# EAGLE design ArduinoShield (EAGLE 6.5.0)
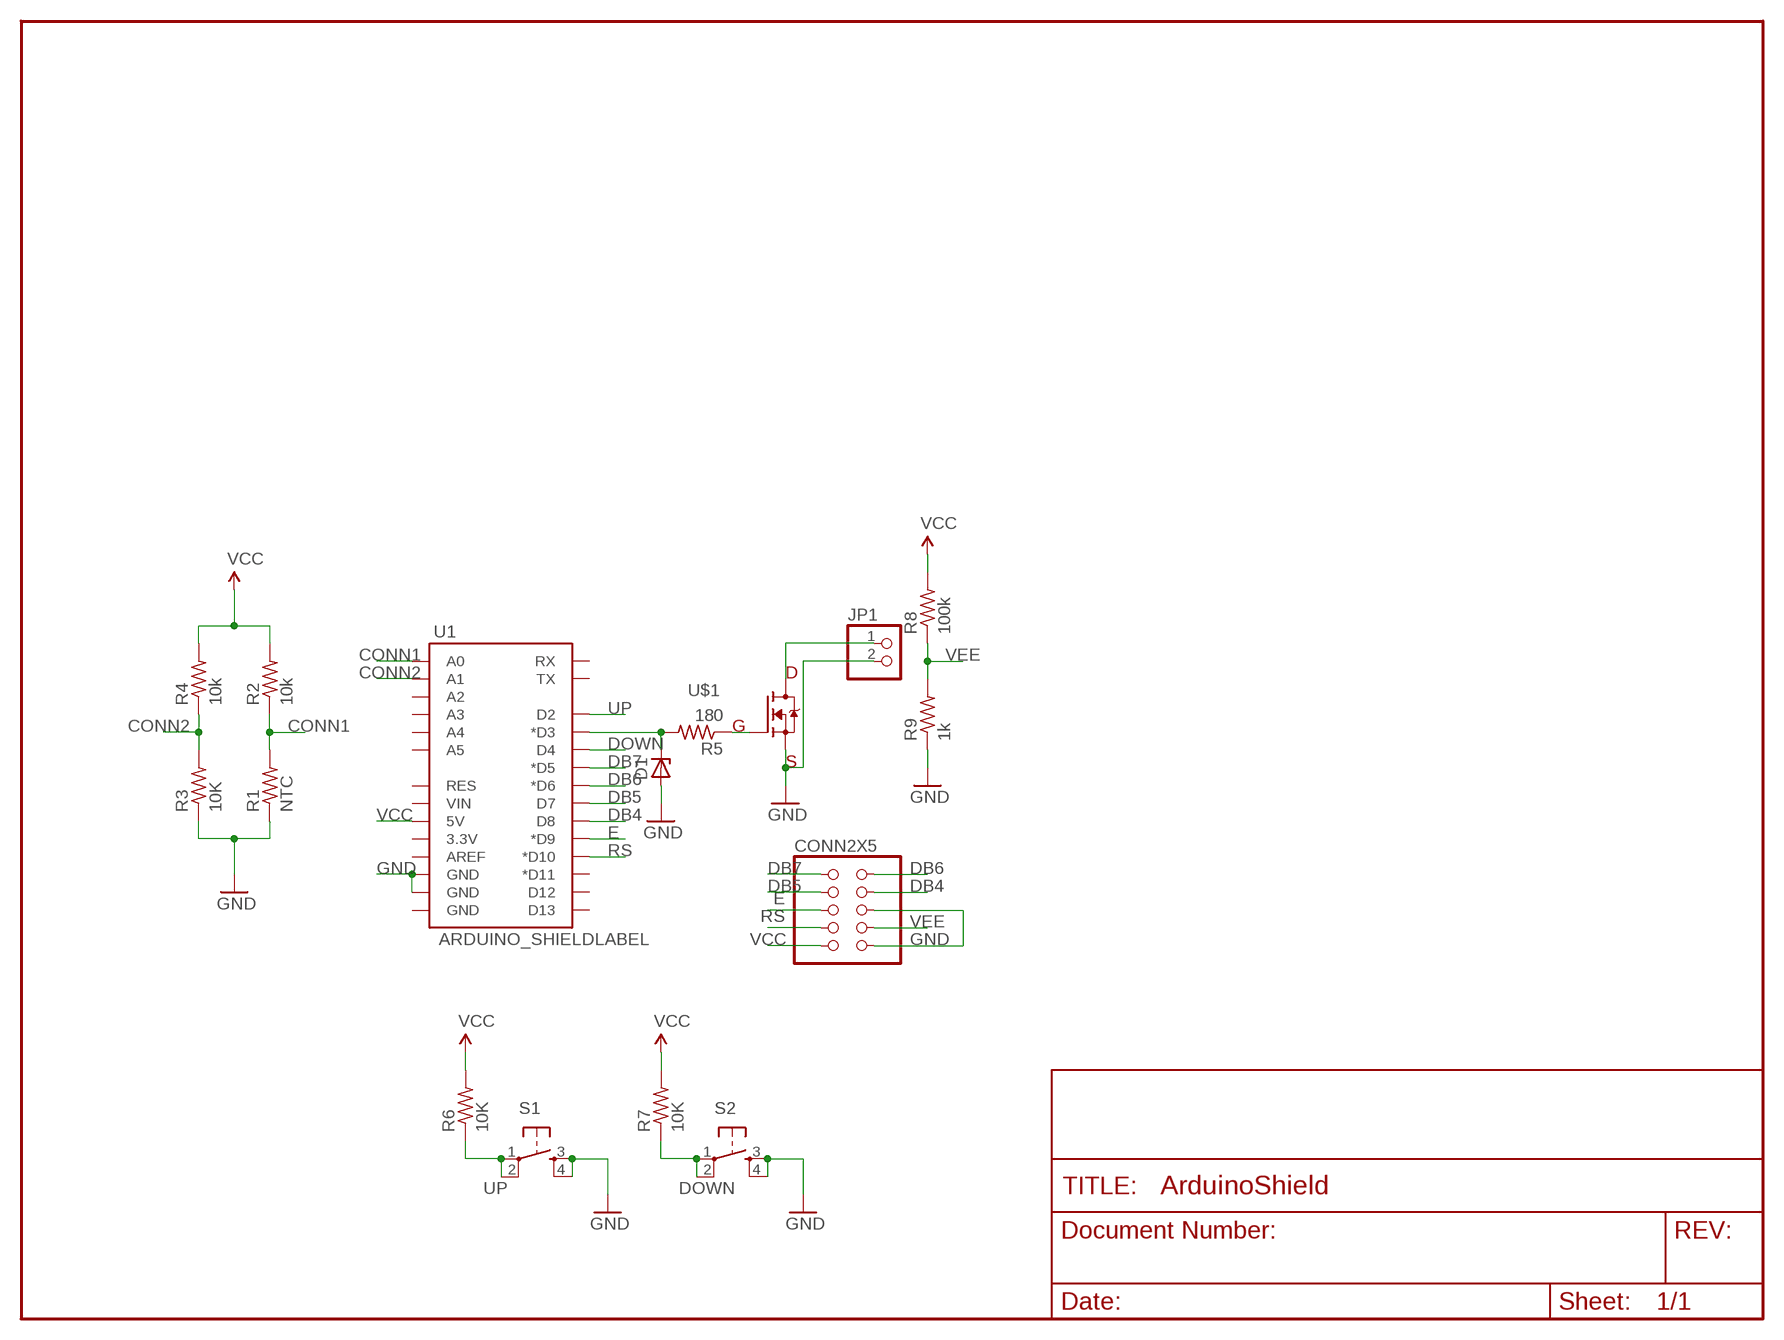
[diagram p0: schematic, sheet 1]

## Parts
CONN2X5  CONN2X05  [2X05SMD]
D1  ZENER_DIODESOD123  [SOD123]
JP1  PINHD-1X2  [1X02]
R1  NTC  RESISTOR1206  [1206]
R2  10k  RESISTOR1206  [1206]
R3  10K  RESISTOR1206  [1206]
R4  10k  RESISTOR1206  [1206]
R5  180  RESISTOR1206  [1206]
R6  10K  RESISTOR1206  [1206]
R7  10K  RESISTOR1206  [1206]
R8  100k  RESISTOR1206  [1206]
R9  1k  RESISTOR1206  [1206]
S1  6MM_SWITCH6MM_SWITCH  [6MM_SWITCH]
S2  6MM_SWITCH6MM_SWITCH  [6MM_SWITCH]
U1  ARDUINO_SHIELDLABEL  [DUEMILANOVE_SHIELD]
U$1  N-MOSFETTO-252  [N-MOSFET]

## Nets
CONN1: R1.2 R2.1 U1.A0
CONN2: R3.2 R4.1 U1.A1
DB4: CONN2X5.7(DB4) U1.D8
DB5: CONN2X5.8(DB5) U1.D7
DB6: CONN2X5.9(DB6) U1.D6(*D6)
DB7: CONN2X5.10(DB7) U1.D5(*D5)
DOWN: R7.1 S2.1(P) S2.2(P1) U1.D4
E: CONN2X5.6(E) U1.D9(*D9)
GND: CONN2X5.1(GND) CONN2X5.5(R/W) D1.ANODE JP1.2 R1.1 R3.1 R9.1 S1.3(S) S1.4(S1) S2.3(S) S2.4(S1) U1.GND@1(GND) U1.GND@2(GND) U$1.2(S)
N$1: D1.CATHODE R5.2 U1.D3(*D3)
N$2: R5.1 U$1.1(G)
N$3: JP1.1 U$1.3(D)
RS: CONN2X5.4(RS) U1.D10(*D10)
UP: R6.1 S1.1(P) S1.2(P1) U1.D2
VCC: CONN2X5.2(VCC) R2.2 R4.2 R6.2 R7.2 R8.2 U1.5V
VEE: CONN2X5.3(VEE) R8.1 R9.2
Unconnected: U1.3.3V U1.A2 U1.A3 U1.A4 U1.A5 U1.AREF U1.D11(*D11) U1.D12 U1.D13 U1.GND@0(GND) U1.RES U1.RX U1.TX U1.VIN

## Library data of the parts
CONN2X5 = 01_ng:CONN2X05
D1 = 01_ng:ZENER_DIODE: zener diode
JP1 = pinhead:PINHD-1X2: PIN HEADER
R1-R9 = 01_ng:RESISTOR
S1 S2 = 01_ng:6MM_SWITCH: OMRON SWITCH
U1 = 01_SparkFun:ARDUINO_SHIELD
U$1 = 01_Ali:N-MOSFET

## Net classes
0 default: clearance 0.205 mm

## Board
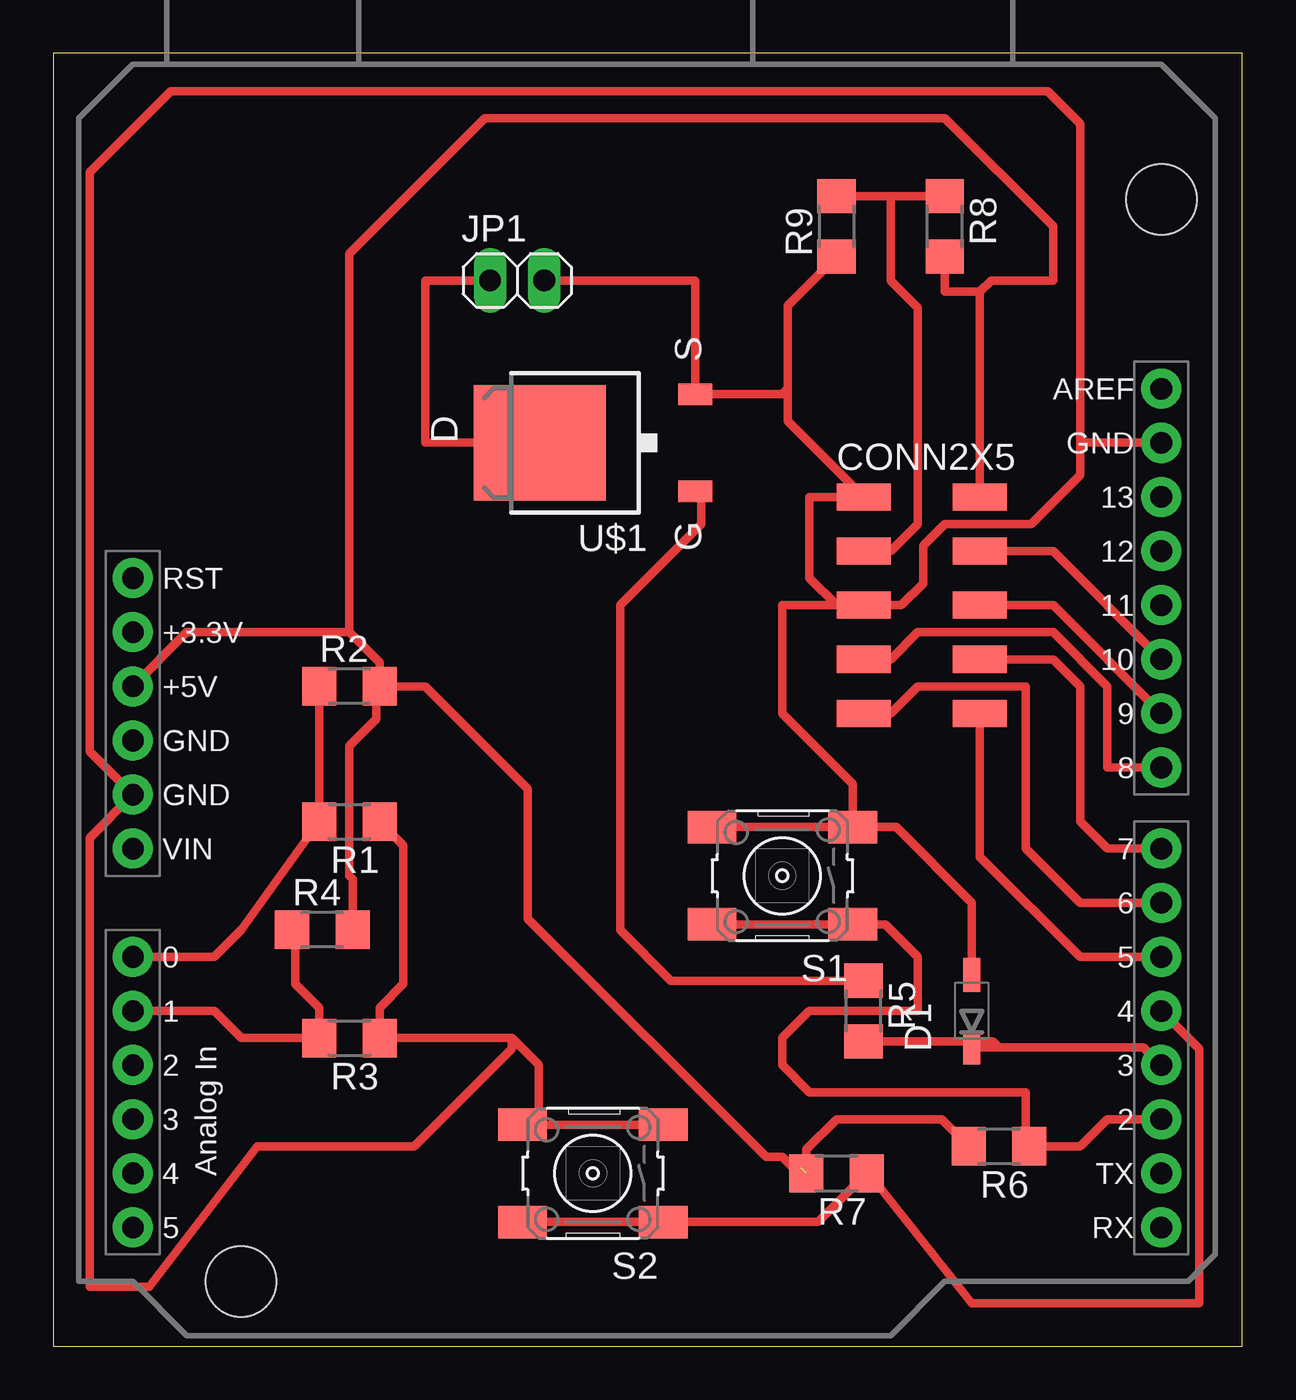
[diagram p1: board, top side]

Size 55.8 x 60.7 mm. Coordinates in mm from the lower left corner, seen from the top.
Outline: 55.8,60.7 0,60.7 0,0 55.8,0 55.8,60.7
Copper layers (1*16): Top 0.035mm / dielectric 1.5mm / Bottom 0.035mm
Design rules "finalProject *": minimum track width 16mil, minimum drill 24mil, track to track 16mil, track to pad 16mil, pad to pad 16mil, via to via 16mil, smd to smd 8mil, copper to edge 40mil, drill to drill 8mil, minimum pad ring 10mil, minimum via ring 8mil, stop-mask expansion 4mil, vias tented up to drill 0mil, thermal gap 10mil

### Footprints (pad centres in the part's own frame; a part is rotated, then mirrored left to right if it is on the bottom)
2X05SMD = smd 2.54 x 1.27: 1 -2.54,3.81; 2 2.92,3.81; 3 -2.54,1.27; 4 2.92,1.27; 5 -2.54,-1.27; 6 2.92,-1.27; 7 -2.54,-3.81; 8 2.92,-3.81; 9 -2.54,-6.35; 10 2.92,-6.35
SOD123 = smd 1.6 x 0.8: ANODE 1.7,0; CATHODE -1.7,0
1X02 = drill 1.016 long: 1 -1.27,0; 2 1.27,0
1206 = smd 1.6 x 1.803: 1 -1.422,0; 2 1.422,0
6MM_SWITCH = smd 2.286 x 1.524: 1 -3.302,2.286; 2 3.302,2.286; 3 -3.302,-2.286; 4 3.302,-2.286
DUEMILANOVE_SHIELD = drill 1.016 pad 1.88: 3.3V 50.8,26.67; 5V 50.8,29.21; A0 50.8,41.91; A1 50.8,44.45; A2 50.8,46.99; A3 50.8,49.53; A4 50.8,52.07; A5 50.8,54.61; AREF 2.54,15.24; D2 2.54,49.53; D3 2.54,46.99; D4 2.54,44.45; D5 2.54,41.91; D6 2.54,39.37; D7 2.54,36.83; D8 2.54,33.02; D9 2.54,30.48; D10 2.54,27.94; D11 2.54,25.4; D12 2.54,22.86; D13 2.54,20.32; GND@0 50.8,31.75; GND@1 50.8,34.29; GND@2 2.54,17.78; RES 50.8,24.13; RX 2.54,54.61; TX 2.54,52.07; VIN 50.8,36.83 | hole 3.302: 45.72,57.15; 2.54,6.35
N-MOSFET = smd 1 x 1.6: 1 -2.28,-4.8; 2 2.28,-4.8 | smd 5.4 x 6.2: 3 0,2.5

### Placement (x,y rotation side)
CONN2X5  40.56,36.06 0 top
D1  43.1,15.74 90 top
JP1  21.77,50.03 0 top
R1  13.89,24.63 180 top
R2  13.89,30.98 0 top
R3  13.89,14.47 180 top
R4  12.62,19.55 0 top
R5  38.02,15.74 270 top
R6  44.37,9.39 180 top
R7  36.75,8.12 180 top
R8  41.83,52.57 270 top
R9  36.75,52.57 90 top
S1  34.21,22.09 180 top
S2  25.32,8.12 180 top
U1  54.53,60.19 180 top
U$1  25.32,42.41 90 top

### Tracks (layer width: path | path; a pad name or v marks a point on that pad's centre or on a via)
CONN1
  Top 0.406: R1.2 8.81,19.55 7.54,18.28 U1.A0 | R1.2 R2.1 | R1.2 12.47,25.75
CONN2
  Top 0.406: U1.A1 7.54,15.74 8.81,14.47 R3.2 12.47,15.89 11.35,17.01 11.35,19.4 R4.1
DB4
  Top 0.406: CONN2X5.7 39.29,32.25 40.56,33.52 46.91,33.52 49.45,30.98 49.45,27.17 U1.D8
DB5
  Top 0.406: CONN2X5.8 46.91,32.25 48.18,30.98 48.18,24.63 49.45,23.36 U1.D7
DB6
  Top 0.406: CONN2X5.9 39.29,29.71 40.56,30.98 45.64,30.98 45.64,23.36 48.18,20.82 U1.D6
DB7
  Top 0.406: CONN2X5.10 43.48,22.98 48.18,18.28 U1.D5
DOWN
  Top 0.406: 53.26,14.47 U1.D4 53.77,13.96 53.77,2.02 43.1,2.02 38.28,8.12 R7.1 35.89,5.83 S2.1 S2.2
E
  Top 0.406: CONN2X5.6 46.91,34.79 U1.D9
GND
  Top 0.406: S2.3 S2.4 22.28,10.66 22.78,10.66 22.78,13.2 21.51,14.47 | 34.47,44.95 34.47,43.42 CONN2X5.1 35.48,39.87 35.48,36.06 36.75,34.79 CONN2X5.5 | 34.47,44.95 34.47,48.86 R9.1 | S1.3 39.55,24.37 43.1,20.82 D1.ANODE | S1.3 37.52,26.41 34.21,29.71 34.21,34.79 CONN2X5.5 | S1.4 S1.3 | 34.47,44.95 34.21,44.69 U$1.2 30.12,50.03 JP1.2 | 21.51,14.47 R3.1 15.32,15.89 16.43,17.01 16.43,23.51 R1.1 | 21.51,14.47 21.51,13.96 16.94,9.39 9.58,9.39 4.5,2.78 1.7,2.78 1.7,23.87 U1.GND@1 1.7,27.93 1.7,55.11 5.51,58.92 46.66,58.92 48.18,57.39 48.18,42.41 | U1.GND@2 48.18,42.41 | 48.18,42.41 48.18,40.88 45.9,38.6 41.83,38.6 40.82,37.58 40.82,35.8 39.8,34.79 CONN2X5.5
N$1
  Top 0.406: D1.CATHODE 44.37,14.04 | 44.37,14.04 51.15,14.04 U1.D3 | R5.2 44.1,14.32 44.37,14.04
N$2
  Top 0.406: R5.1 28.98,17.16 26.59,19.55 26.59,34.79 30.4,38.6 30.4,39.85 U$1.1
N$3
  Top 0.406: U$1.3 17.45,42.41 17.45,50.03 JP1.1
RS
  Top 0.406: CONN2X5.4 46.91,37.33 U1.D10
UP
  Top 0.406: S1.2 S1.1 | U1.D2 49.45,10.66 48.18,9.39 R6.1 45.64,9.54 45.64,11.93 35.48,11.93 34.21,13.2 34.21,14.47 35.48,15.74 40.56,15.74 40.56,18.28 39.04,19.8 S1.1 | S1.1 37.52,19.88 37.42,19.97
VCC  (1 unrouted)
  Top 0.406: CONN2X5.2 43.48,49.5 | R6.2 41.68,10.66 36.75,10.66 35.33,9.24 35.33,8.63 35.08,8.37 34.72,8.37 34.21,8.88 33.45,8.88 22.28,20.06 22.28,26.15 17.45,30.98 R2.2 | R2.2 15.32,32.1 13.89,33.52 | 13.89,33.52 6.27,33.52 U1.5V | 13.89,33.52 13.89,51.3 20.24,57.65 41.83,57.65 46.91,52.57 46.91,50.03 44.02,50.03 43.48,49.5 | R4.2 14.05,21.94 13.89,22.09 13.89,28.18 15.16,29.45 15.16,30.83 R2.2 | 43.48,49.5 41.83,49.5 R8.2
VEE
  Top 0.406: R8.1 39.29,53.99 | 39.29,53.99 36.91,53.99 | 36.91,53.99 36.75,53.84 | R9.2 36.91,53.99 | CONN2X5.3 39.29,37.33 40.56,38.6 40.56,48.76 39.29,50.03 39.29,53.99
